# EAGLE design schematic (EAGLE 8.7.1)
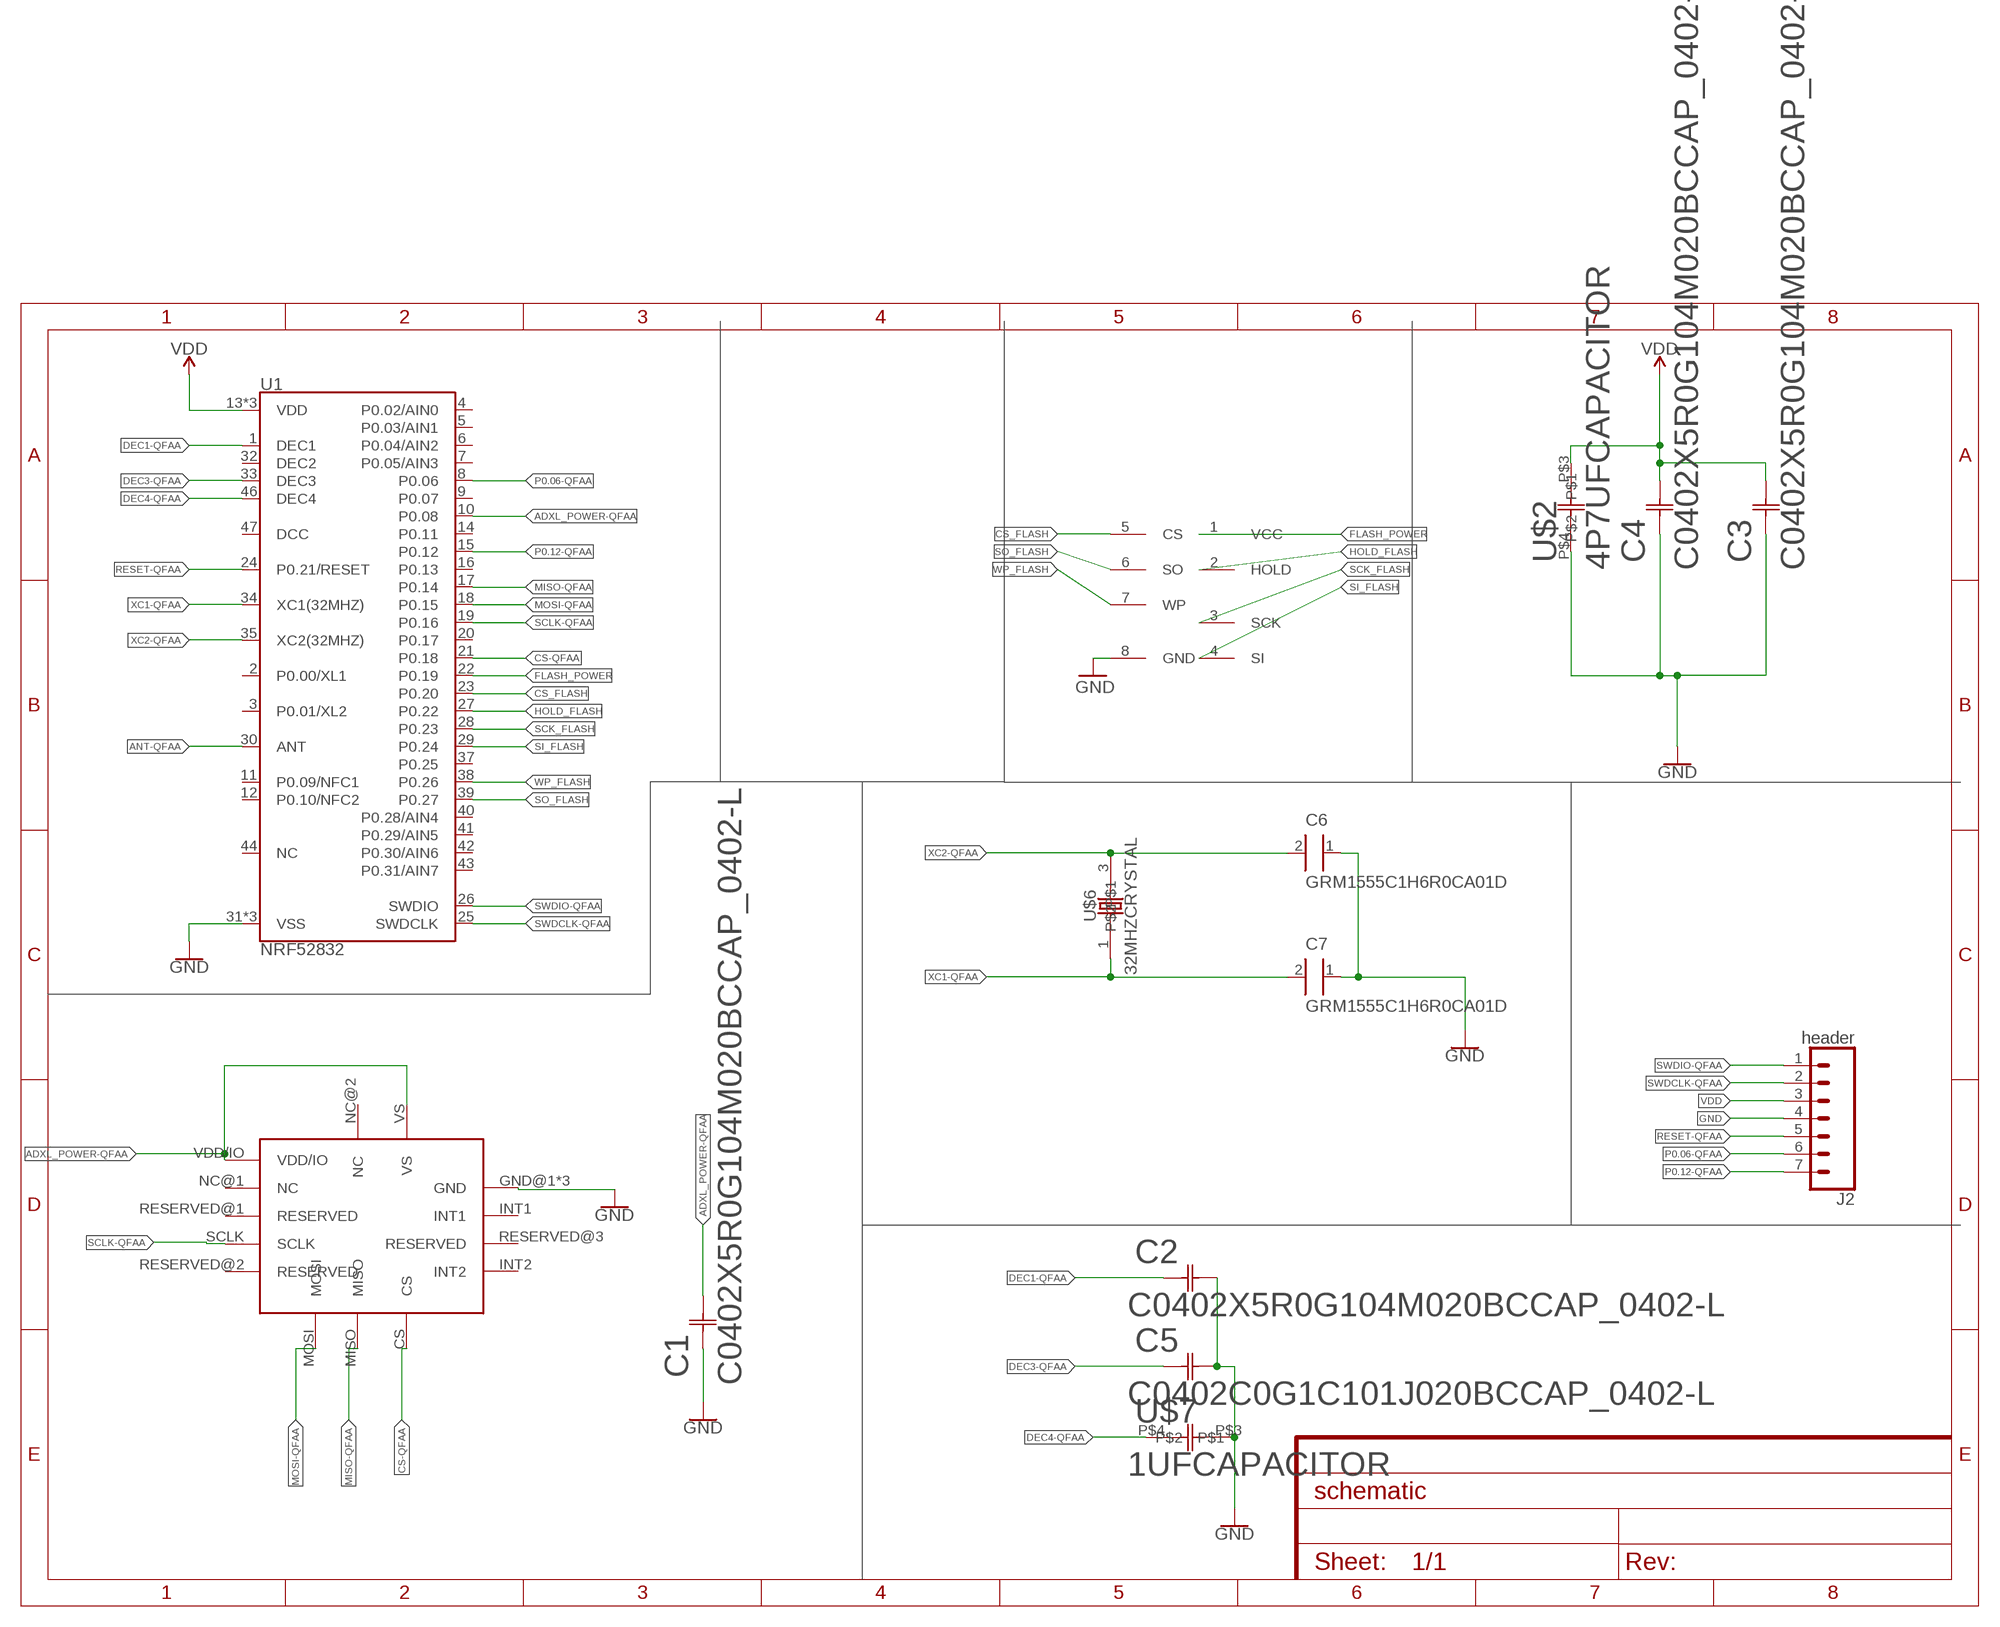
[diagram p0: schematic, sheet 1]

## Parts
C1  C0402X5R0G104M020BCCAP_0402-L  [CAP_0402-L]
C2  C0402X5R0G104M020BCCAP_0402-L  [CAP_0402-L]
C3  C0402X5R0G104M020BCCAP_0402-L  [CAP_0402-L]
C4  C0402X5R0G104M020BCCAP_0402-L  [CAP_0402-L]
C5  C0402C0G1C101J020BCCAP_0402-L  [CAP_0402-L]
C6  GRM1555C1H6R0CA01D  [CAPC1005X55N]
C7  GRM1555C1H6R0CA01D  [CAPC1005X55N]
J2  header  CONN_07  [1X07]
U1  NRF52832  [QFN48-6X6MM]
U$1  ADXL362  [TFLGA-16/3.3MMX3.1MM]
U$2  4P7UFCAPACITOR  [4P7UFCAPACITOR]
U$3  AT25SF161-UUD-T  [AT25SF161-UUD-T]
U$6  32MHZCRYSTAL  [32MHZCRYSTAL]
U$7  1UFCAPACITOR  [1UFCAPACITOR]

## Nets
ADXL_POWER-QFAA: C1.2 U1.10(P0.08) U$1.VDD/IO U$1.VS
ANT-QFAA: U1.30(ANT)
CS-QFAA: U1.21(P0.18) U$1.CS
CS_FLASH: U1.23(P0.20) U$3.5(CS)
DEC1-QFAA: C2.1 U1.1(DEC1)
DEC3-QFAA: C5.1 U1.33(DEC3)
DEC4-QFAA: U1.46(DEC4) U$7.P$4
FLASH_POWER: U1.22(P0.19) U$3.1(VCC)
GND: C1.1 C2.2 C3.1 C4.1 C5.2 C6.1 C7.1 J2.4 U1.31(VSS) U1.45(VSS) U1.EP(VSS) U$1.GND@1(GND) U$1.GND@2(GND) U$1.GND@3(GND) U$2.P$4 U$3.8(GND) U$7.P$3
HOLD_FLASH: U1.27(P0.22) U$3.2(HOLD)
MISO-QFAA: U1.17(P0.14) U$1.MISO
MOSI-QFAA: U1.18(P0.15) U$1.MOSI
P0.06-QFAA: J2.6 U1.8(P0.06)
P0.12-QFAA: J2.7 U1.15(P0.12)
RESET-QFAA: J2.5 U1.24(P0.21/RESET)
SCK_FLASH: U1.28(P0.23) U$3.3(SCK)
SCLK-QFAA: U1.19(P0.16) U$1.SCLK
SI_FLASH: U1.29(P0.24) U$3.4(SI)
SO_FLASH: U1.39(P0.27) U$3.6(SO)
SWDCLK-QFAA: J2.2 U1.25(SWDCLK)
SWDIO-QFAA: J2.1 U1.26(SWDIO)
VDD: C3.2 C4.2 J2.3 U1.13(VDD) U1.36(VDD) U1.48(VDD) U$2.P$3
WP_FLASH: U1.38(P0.26) U$3.7(WP)
XC1-QFAA: C7.2 U1.34(XC1(32MHZ)) U$6.1
XC2-QFAA: C6.2 U1.35(XC2(32MHZ)) U$6.3
Unconnected: U1.2(P0.00/XL1) U1.3(P0.01/XL2) U1.4(P0.02/AIN0) U1.5(P0.03/AIN1) U1.6(P0.04/AIN2) U1.7(P0.05/AIN3) U1.9(P0.07) U1.11(P0.09/NFC1) U1.12(P0.10/NFC2) U1.14(P0.11) U1.16(P0.13) U1.20(P0.17) U1.32(DEC2) U1.37(P0.25) U1.40(P0.28/AIN4) U1.41(P0.29/AIN5) U1.42(P0.30/AIN6) U1.43(P0.31/AIN7) U1.44(NC) U1.47(DCC) U$1.INT1 U$1.INT2 U$1.NC@1(NC) U$1.NC@2(NC) U$1.RESERVED@1(RESERVED) U$1.RESERVED@2(RESERVED) U$1.RESERVED@3(RESERVED)

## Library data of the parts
C1-C4 = 0p1_uF_capacitor:C0402X5R0G104M020BC; MANUFACTURER_PART_NUMBER: C0402C0G1C101J020BC; VENDOR: TDK
C5 = 100_pF_capacitor:C0402C0G1C101J020BC; MANUFACTURER_PART_NUMBER: C0402C0G1C101J020BC; VENDOR: TDK
C6 C7 = 6pf_capacitor_new-bigger:GRM1555C1H6R0CA01D: Cap Ceramic 6pF 50V C0G 0.25pF Pad SMD 0402 125C T/R; DESCRIPTION: 0402 6 pF 50 V ±0.25 pF Tolerance C0G SMT Multilayer Ceramic Capacitor; DIGI-KEY_PART_NUMBER: 490-8222-1-ND; DIGI-KEY_PURCHASE_URL: https://www.digikey.com/product-detail/en/murata-electronics-north-america/GRM1555C1H6R0CA01D/490-8222-1-ND/4380516?WT.z_cid=ref_snapeda&utm_source=snapeda&utm_medium=aggregator&utm_campaign=buynow; MF: Murata; MP: GRM1555C1H6R0CA01D; PACKAGE: 0402 Murata
J2 = SparkFun-Connectors:CONN_07: Multi connection point. Often used as Generic Header-pin footprint for 0.1 inch spaced/style header connections On any of the 0.1 inch spaced packages, you can populate with these: Break Away Headers - Straight (PRT-00116) Break Away Male Headers - Right Angle (PRT-00553) Female Headers (PRT-00115)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
U1 = nrf52832-breakout-temp:NRF52832: Nordic nRF52832 Bluetooth Smart/ANT/2.4GHz RF SoC The nRF52832 SoC is a powerful, highly flexible ultra-low power multiprotocol SoC ideally suited for Bluetooth® Smart ANT and 2.4GHz ultra low-power wireless applications. The nRF52832 SoC is built around a 32-bit ARM® Cortex™-M4F CPU with 512kB +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; PROD_ID: IC-13460
U$1 = ADXL362:ADXL362
U$2 = 4p7_uF_capacitor:4P7UFCAPACITOR
U$3 = AT25SF161-UUD-T:AT25SF161-UUD-T
U$6 = 32_mhz_crystal:32MHZCRYSTAL
U$7 = 1_uF_capacitor:1UFCAPACITOR

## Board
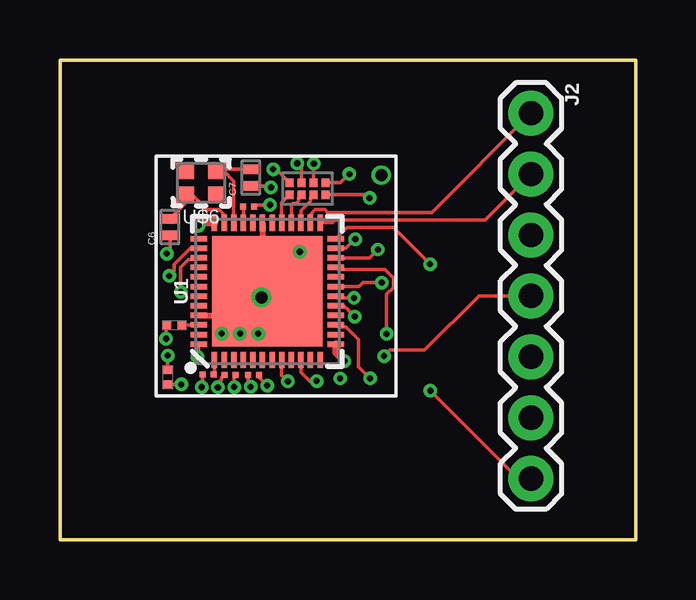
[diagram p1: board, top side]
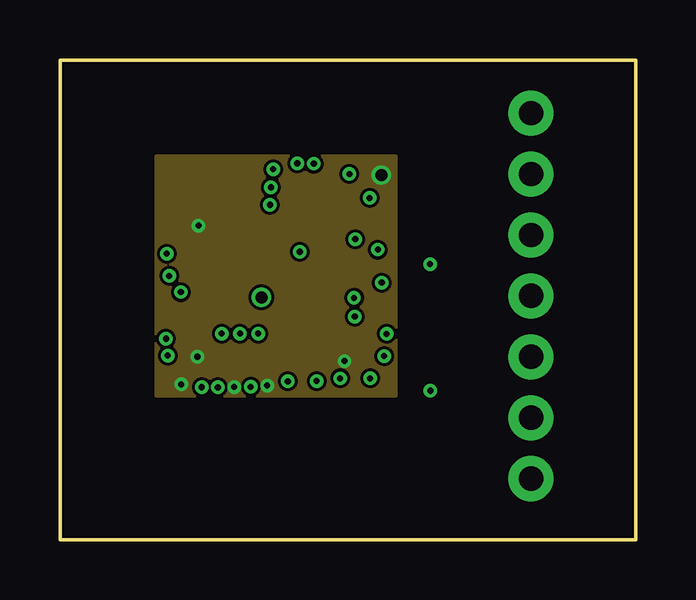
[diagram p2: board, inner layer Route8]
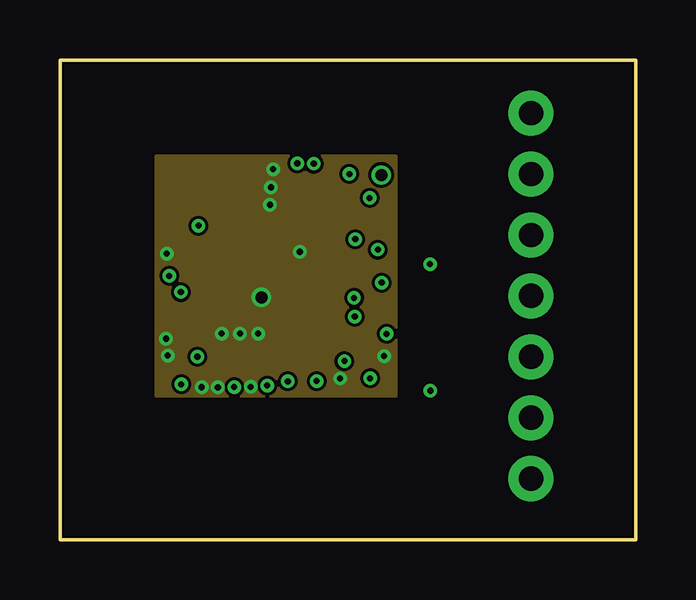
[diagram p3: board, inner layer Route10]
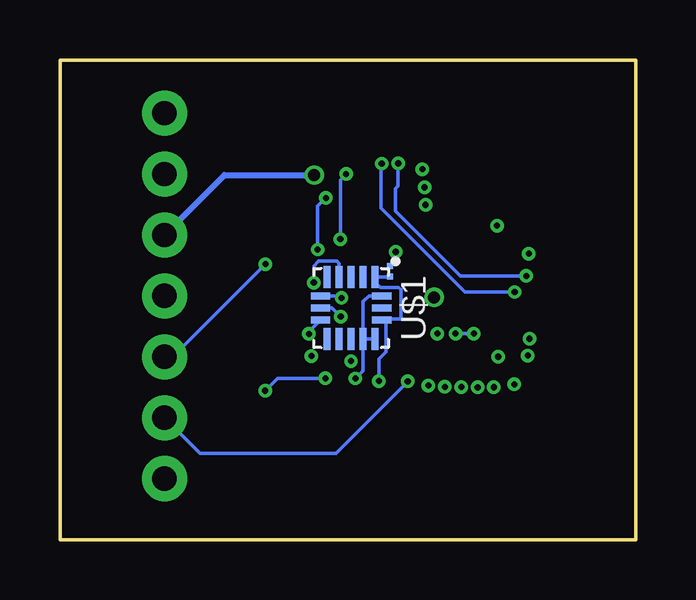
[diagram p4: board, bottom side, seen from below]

Size 24 x 20 mm. Coordinates in mm from the lower left corner, seen from the top.
Outline: 0,0 24,0 24,20 0,20 0,0
Copper layers (1*8*10*16): Top 0.035mm / dielectric 0.42mm / Route8 0.035mm / dielectric 0.62mm / Route10 0.035mm / dielectric 0.42mm / Bottom 0.035mm
Design rules "default *": minimum track width 6mil, minimum drill 10mil, track to track 5mil, track to pad 5mil, pad to pad 5mil, via to via 5mil, smd to smd 2mil, copper to edge 40mil, drill to drill 6mil, minimum pad ring 10mil, minimum via ring 6mil, stop-mask expansion 4mil, vias tented up to drill 0mil, thermal gap 10mil

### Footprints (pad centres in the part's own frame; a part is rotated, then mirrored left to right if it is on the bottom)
CAP_0402-L = smd 0.25 x 0.25: 1 -0.229,0; 2 0.229,0
CAPC1005X55N = smd 0.4 x 0.6: 1 -0.4,0; 2 0.3,0
1X07 = drill 1.016 pad 1.88: 1 0,0; 2 2.54,0; 3 5.08,0; 4 7.62,0; 5 10.16,0; 6 12.7,0; 7 15.24,0
QFN48-6X6MM = smd 0.68 x 0.23: 1 -2.86,2.2; 2 -2.86,1.8; 3 -2.86,1.4; 4 -2.86,1; 5 -2.86,0.6; 6 -2.86,0.2; 7 -2.86,-0.2; 8 -2.86,-0.6; 9 -2.86,-1; 10 -2.86,-1.4; 11 -2.86,-1.8; 12 -2.86,-2.2; 25 2.86,-2.2; 26 2.86,-1.8; 27 2.86,-1.4; 28 2.86,-1; 29 2.86,-0.6; 30 2.86,-0.2; 31 2.86,0.2; 32 2.86,0.6; 33 2.86,1; 34 2.86,1.4; 35 2.86,1.8; 36 2.86,2.2 | smd 0.23 x 0.68: 13 -2.2,-2.86; 14 -1.8,-2.86; 15 -1.4,-2.86; 16 -1,-2.86; 17 -0.6,-2.86; 18 -0.2,-2.86; 19 0.2,-2.86; 20 0.6,-2.86; 21 1,-2.86; 22 1.4,-2.86; 23 1.8,-2.86; 24 2.2,-2.86; 37 2.2,2.86; 38 1.8,2.86; 39 1.4,2.86; 40 1,2.86; 41 0.6,2.86; 42 0.2,2.86; 43 -0.2,2.86; 44 -0.6,2.86; 45 -1,2.86; 46 -1.4,2.86; 47 -1.8,2.86; 48 -2.2,2.86 | smd 4.6 x 4.6: EP 0,0
TFLGA-16/3.3MMX3.1MM = smd 0.3 x 0.8: CS 0.5,-1.275; GND@3 -0.5,1.275; MISO 0,-1.275; MOSI -0.5,-1.275; NC@2 0,1.275; VS 0.5,1.275 | smd 0.925 x 0.3: GND@1 1.288,0.5; GND@2 1.288,1; INT1 1.288,0; INT2 1.288,-1; NC@1 -1.288,0.5; RESERVED@1 -1.288,0; RESERVED@2 -1.288,-1; RESERVED@3 1.288,-0.5; SCLK -1.288,-0.5; VDD/IO -1.288,1
4P7UFCAPACITOR = smd 0.35 x 0.4: P$3 0.18,0.15; P$4 0.8,0.15
AT25SF161-UUD-T = smd 0.35 x 0.35: 1 1.2,0.9; 2 1.2,0.4; 3 1.2,-0.1; 4 1.2,-0.6; 5 0.7,0.9; 6 0.7,0.4; 7 0.7,-0.1; 8 0.7,-0.6
32MHZCRYSTAL = smd 0.75 x 0.7: 1 0.485,0.47; 2 1.835,0.47; 3 1.835,1.47; 4 0.485,1.47
1UFCAPACITOR = smd 0.35 x 0.4: P$3 0.18,0.15; P$4 0.8,0.15

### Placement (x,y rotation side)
C1  10.24,11.19 270 bottom
C2  6.19,6.88 180 top
C3  8.07,6.87 0 top
C4  7.09,6.87 0 top
C5  7.86,13.88 0 top
C6  4.59,13.08 90 top
C7  7.96,15.14 90 top
J2  19.64,17.78 270 top
U1  8.65,10.35 90 top
U$1  11.86,9.66 270 bottom
U$2  4.65,6.28 90 top
U$3  10.17,15.58 270 top
U$6  7.05,15.85 180 top
U$7  4.27,8.79 0 top

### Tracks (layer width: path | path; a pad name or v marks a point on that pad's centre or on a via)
ADXL_POWER-QFAA  (via drill 0.25)
  Top 0.152: U1.10 10.05,6.96 10.4,6.61 v10.71,6.61
  Bottom 0.152: C1.2 10.25,10.94 U$1.VDD/IO 10.86,10.72 10.64,10.51 9.88,10.51 9.79,10.42 9.79,9.2 10.4,9.2 | 10.4,9.2 10.54,9.2 U$1.VS | v10.71,6.61 10.71,7.52 10.4,7.83 10.4,9.2
CS-QFAA  (via drill 0.25 pad 0.46)
  Top 0.152: U1.21 11.59,11.27 13.54,11.27 13.9,10.91 13.9,10.51 13.62,10.23 v13.62,8.57
  Bottom 0.152: v13.62,8.57 13.62,8.67 U$1.CS
CS_FLASH  (via drill 0.25 pad 0.46)
  Top 0.152: U1.23 11.93,12.15 v12.31,12.53 | v12.07,15.24 11.71,14.88 U$3.5
  Bottom 0.152: v12.31,12.53 12.31,15 v12.07,15.24
DEC1-QFAA
  Top 0.152: C2.1 6.45,6.91 U1.1
DEC3-QFAA
  Top 0.152: U1.33 7.65,13.87 C5.1
DEC4-QFAA
  Top 0.152: U$7.P$4 5.78,8.94 U1.46
FLASH_POWER  (via drill 0.25 pad 0.46)
  Top 0.152: U$3.1 12.78,14.38 v12.91,14.24 | v13.25,12.09 12.91,11.75 U1.22
  Bottom 0.152: v12.91,14.24 13.25,13.9 v13.25,12.09
GND  (via drill 0.25, 0.25 pad 0.46, 0.25 pad 0.51, 0.5 pad 0.46)
  Top 0.152: U$7.P$3 4.42,8.91 v4.42,8.38 | U$2.P$4 v4.5,7.67 | v13.52,7.65 13.76,7.9 15.2,7.9 17.46,10.16 J2.4 | 8.41,10.12 8.45,10.15 8.45,10.55 U1.EP v8.4,10.1 | v8.4,10.1 6.89,8.59 v6.74,8.59 | v7.5,8.59 v8.27,8.59 | C3.1 7.84,6.48 v7.95,6.37 | C4.1 6.74,6.76 6.74,6.67 6.58,6.51 v6.58,6.35 | C2.2 5.96,6.4 v5.91,6.35 | C5.2 8.17,13.96 v8.75,13.96 | C7.1 8.74,14.74 v8.8,14.69 | U$3.8 9.01,15.45 v8.89,15.45 | C6.1 4.59,12.05 v4.46,11.92 | 8.45,12.5 8.4,12.45 v8.4,10.1
  Top 0.254: U1.31 8.45,12.5 8.45,10.55 | U1.45 7.65,9.35 v8.4,10.1 8.41,10.12 U1.EP
  Bottom 0.152: C1.1 10,11.65 v10,12 | U$1.GND@2 U$1.GND@1 | U$1.GND@1 11.36,7.04 v11.68,6.72 | v6.74,8.59 v7.5,8.59 | U$1.GND@1 11.36,9.92 11.12,10.16 U$1.GND@3
  pour Route10: 4,16 4,6 14,6 14,16
HOLD_FLASH
  Top 0.152: U$3.2 10.45,14.26 10.45,14.12 10.05,13.71 U1.27
MISO-QFAA  (via drill 0.25 pad 0.46)
  Top 0.152: v12.29,9.3 12.05,9.54 12.05,9.55 11.85,9.75 U1.17
  Bottom 0.152: v12.29,9.3 12.65,9.66 U$1.MISO
MOSI-QFAA  (via drill 0.25 pad 0.46)
  Top 0.152: U1.18 11.58,10.07 v12.26,10.07
  Bottom 0.152: v12.26,10.07 12.34,10.16 U$1.MOSI
P0.06-QFAA  (via drill 0.25 pad 0.46)
  Top 0.152: U1.8 9.25,6.85 v9.5,6.6
  Bottom 0.152: v9.5,6.6 12.5,3.6 18.16,3.6 J2.6
P0.12-QFAA  (via drill 0.25 pad 0.46)
  Top 0.152: v12.93,6.72 12.45,7.2 12.45,8.35 11.93,8.87 11.59,8.87 U1.15 | v15.44,6.21 19.11,2.54 J2.7
  Bottom 0.152: v12.93,6.72 14.93,6.72 v15.44,6.21
RESET-QFAA  (via drill 0.25)
  Top 0.152: U1.24 11.97,13.01 13.91,13.01 v15.43,11.49
  Bottom 0.152: v15.43,11.49 19.3,7.62 J2.5
SCK_FLASH
  Top 0.152: U1.28 9.65,13.95 9.7,14 9.83,14 9.95,14.12 9.95,14.26 U$3.3
SCLK-QFAA  (via drill 0.25 pad 0.46)
  Top 0.152: U1.19 12.05,10.55 12.06,10.56 12.46,10.56 12.47,10.55 12.48,10.55 12.64,10.71 v13.41,10.71
  Bottom 0.152: v13.41,10.71 13.41,11.41 13.22,11.61 12.45,11.61 12.36,11.52 U$1.SCLK
SI_FLASH
  Top 0.152: U1.29 9.25,14.05 U$3.4
SO_FLASH  (via drill 0.25 pad 0.46)
  Top 0.152: U1.39 5.7,11.67 5.36,11.67 5.04,11.35 v5.04,10.32 | v10.58,15.68 10.57,15.67 U$3.6
  Bottom 0.152: v5.04,10.32 7.11,10.32 10.62,13.83 10.62,15.64 v10.58,15.68
SWDCLK-QFAA
  Top 0.152: U1.25 11.36,13.21 11.47,13.32 17.71,13.32 J2.2
SWDIO-QFAA
  Top 0.152: U1.26 10.45,13.56 10.64,13.75 11.04,13.75 11.16,13.64 15.5,13.64 J2.1
VDD  (via drill 0.25, 0.25 pad 0.46, 0.25 pad 0.51, 0.5 pad 0.46)
  Top 0.152: U1.48 5.79,7.68 v5.73,7.62 | U$2.P$3 5.05,6.46 v5.06,6.48 | C3.2 8.29,6.77 v8.64,6.42 | C4.2 7.27,6.83 v7.27,6.36
  Top 0.305: U1.36 5.89,13.21 v5.77,13.09 | U1.13 11.51,7.8 v11.86,7.44
  Route8 0.152: v5.73,7.62 v5.73,7.63
  Bottom 0.254: J2.3 17.14,15.2 v13.4,15.2
  pour Route8: 4,16 14,16 14,6 4,6
WP_FLASH  (via drill 0.25 pad 0.46)
  Top 0.152: v4.56,11 4.76,11.2 4.76,11.47 5.44,12.15 U1.38 | v9.9,15.69 10.07,15.51 U$3.7
  Bottom 0.152: v4.56,11 7.3,11 10,13.7 10,14.64 9.9,14.75 v9.9,15.69
XC1-QFAA
  Top 0.152: C7.2 6.63,15.44 U$6.1 6.81,15.38 7.25,14.95 U1.34
XC2-QFAA
  Top 0.152: U1.35 6.8,13.25 6.8,13.6 6.64,13.75 6.13,13.75 5.51,14.38 U$6.3 5.21,14.01 C6.2

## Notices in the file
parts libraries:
SparkFun-Aesthetics: Licensing: Creative Commons ShareAlike 4.0 International - https://creativecommons.org/licenses/by-sa/4.0
